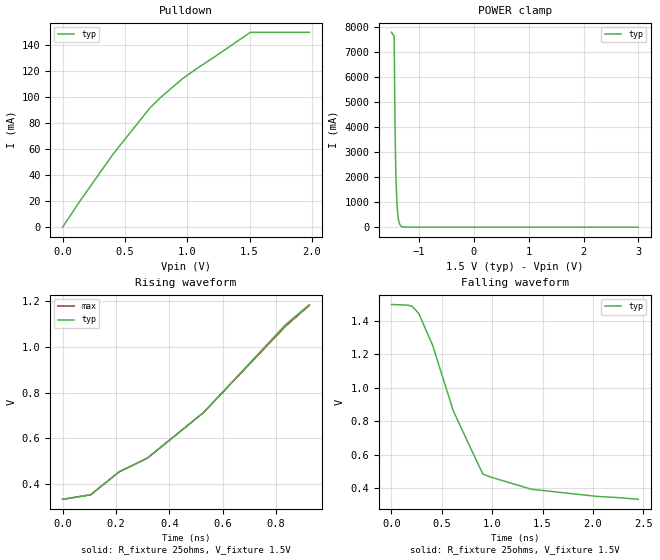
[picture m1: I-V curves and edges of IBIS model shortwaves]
[IBIS Ver]   2.1
[File Name]   bug47.ibs
[File Rev]   0.1
[Source]
[Date]   9/20/2000
[Comment char]  |_char
[Disclaimer] This IBIS file demonstrates an IBIS parser flaw, and is not
   intended to be representative of any known component.
[Component]   shortwaves
[Manufacturer]  Cadence Design Systems
[Package]
| variable   typ   min   max
R_pkg   0ohms   NA   NA
L_pkg   0H   NA   NA
C_pkg   0F   NA   NA
[Pin]   signal_name   model_name   R_pin   L_pin   C_pin
1   1   shortwaves
| Models and submodels in the file (1): shortwaves (I/O_open_drain)
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[Model] shortwaves
Model_type  I/O_open_drain
Polarity   Non-Inverting
Enable   Active-Low
Vinl = 0.9
Vinh = 1.1
Vmeas = 1.00
Cref  = 0.00p
Rref  = 25.00
Vref  = 1.50
| variable   typ   min   max
C_comp   3.28pF  NA   NA
[Voltage Range] 1.5V   NA   NA
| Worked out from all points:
|   slope of the pulldown table from 0 to 0.225 V, typ, clamps not added: 7.08 ohm
|   POWER clamp passes 1 mA (typ) near -1.23 V on its own axis
|   rising waveform, R_fixture 25ohms, V_fixture 1.5V: 20-80 % time 469ps typ, NA min, 472ps max; typ from 0.334 V to 1.18 V
|   falling waveform, R_fixture 25ohms, V_fixture 1.5V: 20-80 % time 442ps typ, NA min, NA max; typ from 1.5 V to 0.334 V
[POWER Clamp]
|Voltage   I(typ)  I(min)  I(max)   Table is VCC relative
-1.5V     7.8A       NA         NA
-1.45V    7.64A      NA         NA
-1.443V   5.72A      NA         NA
-1.437V   4.46A      NA         NA
-1.431V   3.48A      NA         NA
-1.425V   2.71A      NA         NA
-1.418V   2.03A      NA         NA
-1.4V     960mA      NA         NA
-1.387V   560mA      NA         NA
-1.372V   300mA      NA         NA
-1.327V   47mA       NA         NA
2.998V    0A         NA         NA
[Pullup]
|Voltage   I(typ)  I(min)  I(max)   Table is VCC relative
-481mV    0A         NA         0A
-480mV    0A         NA         0A
1.499V    0A         NA         0A
[Pulldown]
|Voltage   I(typ)  I(min)  I(max)
0V        0A         NA         NA
150mV     21.59mA    NA         NA
406mV     56.34mA    NA         NA
699mV     91.6mA     NA         NA
788mV     100mA      NA         NA
962mV     114.3mA    NA         NA
1.07V     121.6mA    NA         NA
1.237V    132.3mA    NA         NA
1.507V    150mA      NA         NA
1.981V    150mA      NA         NA
[Ramp]
| variable   typ   min   max
dV/dt_r 698.4mV/888ps   NA   NA
dV/dt_f 698.4mV/1.47ns  NA   NA
R_load = 25ohms
[Rising Waveform]
R_fixture = 25ohms
V_fixture = 1.5V
V_fixture_max = 1.6V
|Time   V(typ)  V(min)  V(max)
0s        334.2mV    NA         334.1mV
105ps     354mV      NA         354mV
212ps     454.1mV    NA         454.1mV
317ps     513.4mV    NA         513.4mV
528ps     712.5mV    NA         712.5mV
836ps     1.097V     NA         1.09V
925ps     1.184V     NA         1.18V
||| Points have been removed from the [Rising Waveform], resulting in
||| a waveform that does not end at 1.5V.
[Falling Waveform]
R_fixture = 25ohms
V_fixture = 1.5V
|Time   V(typ)  V(min)  V(max)
0s        1.498V     NA         NA
159ps     1.495V     NA         NA
203ps     1.488V     NA         NA
270ps     1.446V     NA         NA
409ps     1.254V     NA         NA
613ps     863.8mV    NA         NA
907ps     485.5mV    NA         NA
1.387ns   394.7mV    NA         NA
2.041ns   351.6mV    NA         NA
2.45ns    334.2mV    NA         NA
